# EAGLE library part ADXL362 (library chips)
IC ACCEL DIG LO PWR 3AX 16LGA
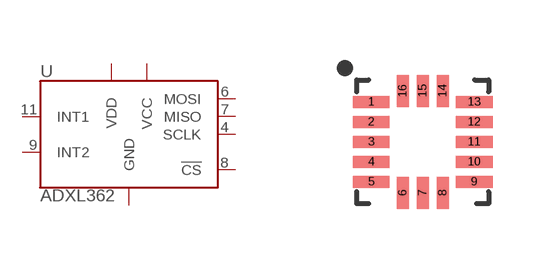
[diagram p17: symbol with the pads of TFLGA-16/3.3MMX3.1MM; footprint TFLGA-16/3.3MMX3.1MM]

Designator prefix U

## ADXL362 (DIGIKEY: ADXL362BCCZ-RL7CT-ND; MOUSER: 584-ADXL362BCCZ-R7; NEWARK: 47W0478)  [TFLGA-16/3.3MMX3.1MM]
1  VDD
4  SCLK
6  MOSI
7  MISO
8  !CS
9  INT2
11  INT1
12  GND
13  GND
14  VCC
16  GND

## Footprint TFLGA-16/3.3MMX3.1MM (pad centres in mm)
smd 0.925 x 0.3: 1 -1.288,1; 2 -1.288,0.5; 3 -1.288,0; 4 -1.288,-0.5; 5 -1.288,-1; 9 1.288,-1; 10 1.288,-0.5; 11 1.288,0; 12 1.288,0.5; 13 1.288,1
smd 0.3 x 0.8: 6 -0.5,-1.275; 7 0,-1.275; 8 0.5,-1.275; 14 0.5,1.275; 15 0,1.275; 16 -0.5,1.275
